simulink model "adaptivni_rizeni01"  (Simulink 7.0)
settings: Solver=ode45  StartTime=0.0  StopTime=50  RelTol=1e-3
libraries: simulink x1

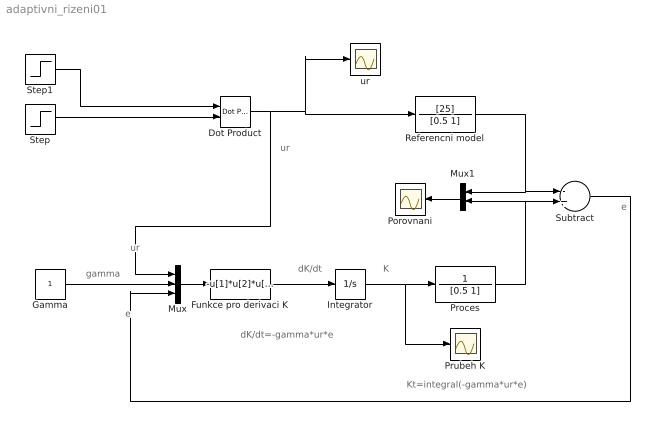
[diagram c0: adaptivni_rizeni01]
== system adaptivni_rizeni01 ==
  note: ur
  note: e
  note: e
  note: dK/dt=-gamma*ur*e
  note: ur
  note: gamma
  note: Kt=integral(-gamma*ur*e)
  note: dK/dt
  note: K
  Dot Product : simulink/Math Operations/Dot Product  InputSameDT=on  OutDataType=sfix(16)  OutScaling=2^-10  DoSatur=off
  Funkce pro derivaci K : Fcn  Expr=-u[1]*u[2]*u[3]
  Gamma : Constant  OutDataType=sfix(16)  OutScaling=2^0
  Integrator : Integrator
  Mux : Mux  Inputs=3
  Mux1 : Mux  Orientation=left  Inputs=2
  Porovnani : Scope
  Proces : TransferFcn  Numerator=1  Denominator=[0.5 1]
  Prubeh K : Scope
  Referencni model : TransferFcn  Numerator=[25]  Denominator=[0.5 1]
  Step : Step  Time=0  SampleTime=0
  Step1 : Step  Time=25  Before=1  After=2  SampleTime=0
  Subtract : Sum  Inputs=-+  OutDataType=sfix(16)  OutScaling=2^-10
  ur : Scope
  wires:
  Step/1 -> Dot Product/2
  Mux/1 -> Funkce pro derivaci K/1
  Subtract/1 -> Mux/3
  Funkce pro derivaci K/1 -> Integrator/1
  Integrator/1 -> Proces/1, Prubeh K/1
  Gamma/1 -> Mux/2
  Dot Product/1 -> Mux/1, Referencni model/1, ur/1
  Step1/1 -> Dot Product/1
  Referencni model/1 -> Subtract/1, Mux1/1
  Proces/1 -> Subtract/2, Mux1/2
  Mux1/1 -> Porovnani/1
